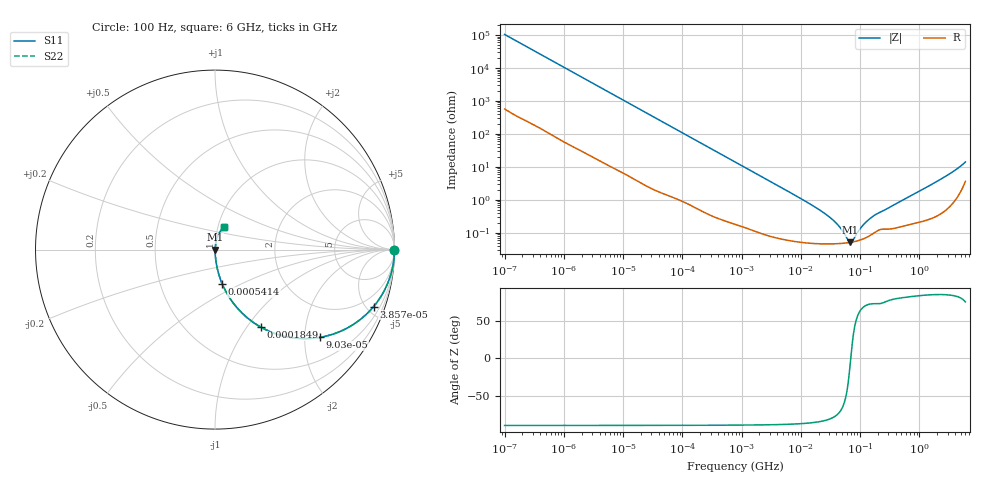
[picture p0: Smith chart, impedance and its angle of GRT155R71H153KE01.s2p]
!Murata Part Number: GRT155R71H153KE01
!These Parameters are Measured in Series Mode Connection
!Data Generated on Jun 19, 2026
!  o--ll--o
!Port1  Port2
!  o------o
!Operation Temp=25[degC], DC Bias Voltage=0[V]
!Freq. Start=100[Hz] Stop=6[GHz] 401[Steps]
# Hz S RI R 50
!Freq.(Hz) S11(Real) S11(Imag) S21(Real) S21(Imag) S12(Real) S12(Imag) S22(Real) S22(Imag)
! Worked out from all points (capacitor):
!   401 points, 100 Hz to 6 GHz, reference 50 ohm
!   read as one part in series: C = 15.2 nF near 109 Hz
!   lowest |Z| = 50.9 mohm at 68.17 MHz (marker M1)
!   series resonance near 69.68 MHz, so ESL is about 340 pH
!   S11 on the Smith chart (normalised r, x): 100 Hz: open; 38.57 kHz: 1.04, -5.54; 90.3 kHz: 1.02, -2.38; 184.9 kHz: 1.01, -1.17; 541.4 kHz: 1.00, -0.40; 6 GHz: 1.07, +0.27
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100  1 -0.000955  6.1e-06 0.000955  6.1e-06 0.000955  1 -0.000955
2008  0.9995 -0.019  0.000467 0.019  0.000467 0.019  0.9995 -0.019
11009  0.9888 -0.1022  0.0112 0.1022  0.0112 0.1022  0.9888 -0.1022
38569  0.8832 -0.318  0.1168 0.318  0.1168 0.318  0.8832 -0.318
40335  0.8738 -0.3289  0.1262 0.3289  0.1262 0.3289  0.8738 -0.3289
90302  0.5846 -0.4887  0.4154 0.4887  0.4154 0.4887  0.5846 -0.4887
184852  0.2554 -0.4317  0.7446 0.4317  0.7446 0.4317  0.2554 -0.4317
302498  0.1153 -0.3147  0.8847 0.3147  0.8847 0.3147  0.1153 -0.3147
541393  0.0404 -0.1914  0.9596 0.1914  0.9596 0.1914  0.0404 -0.1914
774597  0.0209 -0.1369  0.9791 0.1369  0.9791 0.1369  0.0209 -0.1369
2481164  0.00279 -0.0439  0.9972 0.0439  0.9972 0.0439  0.00279 -0.0439
1.555665e7  0.000514 -0.00675  0.9995 0.00675  0.9995 0.00675  0.000514 -0.00675
3.64232e7  0.000461 -0.00221  0.9995 0.00221  0.9995 0.00221  0.000461 -0.00221
4.556224e7  0.000467 -0.00139  0.9995 0.00139  0.9995 0.00139  0.000467 -0.00139
6.233367e7  0.000492 -0.000353  0.9995 0.000353  0.9995 0.000353  0.000492 -0.000353
6.817316e7  0.000504 -6.86e-05  0.9995 6.86e-05  0.9995 6.86e-05  0.000504 -6.86e-05
7.455971e7  0.000518 0.000215  0.9995 -0.000215  0.9995 -0.000215  0.000518 0.000215
1.020051e8  0.0006 0.00123  0.9994 -0.00123  0.9994 -0.00123  0.0006 0.00123
1.395531e8  0.000774 0.00234  0.9992 -0.00234  0.9992 -0.00234  0.000774 0.00234
3.124326e8  0.00131 0.00565  0.9987 -0.00565  0.9987 -0.00565  0.00131 0.00565
2.240541e9  0.00521 0.0403  0.9948 -0.0403  0.9948 -0.0403  0.00521 0.0403
6e9  0.0509 0.124  0.9491 -0.124  0.9491 -0.124  0.0509 0.124
